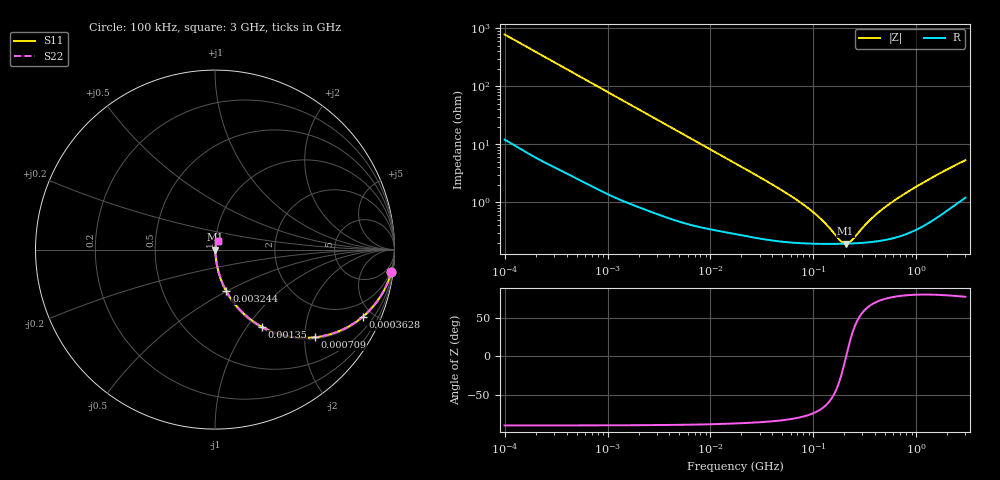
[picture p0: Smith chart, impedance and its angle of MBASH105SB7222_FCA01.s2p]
! MBASH105SB7222_FCA01  S-PARAMETER MODEL  ( Standard Model )
! Model Generated by TAIYO YUDEN Corporation (http://www.ty-top.com)
! Version 1.0
! TAIYO YUDEN Control No. 220601
! Copyright(c) 2019 TAIYO YUDEN CO.,LTD. All Rights Reserved.
! Product Description (link to TY-COMPAS)
! https://ds.yuden.co.jp/TYCOMPAS/or/detail?pn=MBASH105SB7222KFCA01&u=M
! Products Name : Multilayer Ceramic Capacitors
! Characteristics :
!  Capacitance : 2200 [pF] , Rated Voltage : 100 [V] , TCC : X7R
!  Case Size : 1.0 x 0.5 / 0.039 x 0.02 [mm/inch] , Thickness : 0.5 / 0.02 [mm/inch]
!  (Conditions: Temperature = 25 [degC] , DC Bias Voltage = 0 [V])
! External Node Assignments :
!  1  o---| |---o  2
! GND o---------o GND
! Frequency Range : 100kHz  -  3GHz  [ 401 STEP ]
# MHZ S RI R 50
! Freq[MHz].  S11 Real  S11 Imag  S21 Real  S21 Imag  S12 Real  S12 Imag  S22 Real  S22 Imag
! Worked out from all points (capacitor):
!   401 points, 100 kHz to 3 GHz, reference 50 ohm
!   read as one part in series: C = 2.03 nF near 105.3 kHz
!   lowest |Z| = 194 mohm at 205.6 MHz (marker M1)
!   series resonance near 208 MHz, so ESL is about 290 pH
!   S11 on the Smith chart (normalised r, x): 100 kHz: 1, -16; 362.8 kHz: 1.07, -4.36; 709 kHz: 1.04, -2.24; 1.35 MHz: 1.02, -1.18; 3.244 MHz: 1.01, -0.50; 3 GHz: 1.02, +0.10
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0.1  0.982 -0.1255  0.018 0.1255  0.018 0.1255  0.982 -0.1255
0.21115  0.9295 -0.2486  0.0705 0.2486  0.0705 0.2486  0.9295 -0.2486
0.362777  0.822 -0.3747  0.178 0.3747  0.178 0.3747  0.822 -0.3747
0.562235  0.6632 -0.4645  0.3368 0.4645  0.3368 0.4645  0.6632 -0.4645
0.709011  0.5562 -0.4885  0.4438 0.4885  0.4438 0.4885  0.5562 -0.4885
0.965977  0.4069 -0.4827  0.5931 0.4827  0.5931 0.4827  0.4069 -0.4827
1.350433  0.2635 -0.4314  0.7365 0.4314  0.7365 0.4314  0.2635 -0.4314
2.039661  0.1393 -0.336  0.8607 0.336  0.8607 0.336  0.1393 -0.336
3.161081  0.0661 -0.2368  0.9339 0.2368  0.9339 0.2368  0.0661 -0.2368
3.243608  0.0632 -0.2316  0.9368 0.2316  0.9368 0.2316  0.0632 -0.2316
7.027689  0.0169 -0.1132  0.9831 0.1132  0.9831 0.1132  0.0169 -0.1132
17.7727  0.0049 -0.0457  0.9951 0.0457  0.9951 0.0457  0.0049 -0.0457
52.46276  0.00229 -0.0149  0.9977 0.0149  0.9977 0.0149  0.00229 -0.0149
97.38194  0.00198 -0.00671  0.998 0.00671  0.998 0.00671  0.00198 -0.00671
129.3002  0.00193 -0.00397  0.9981 0.00397  0.9981 0.00397  0.00193 -0.00397
180.7614  0.00192 -0.00113  0.9981 0.00113  0.9981 0.00113  0.00192 -0.00113
205.6221  0.00193 -9.07e-05  0.9981 9.07e-05  0.9981 9.07e-05  0.00193 -9.07e-05
233.9019  0.00195 0.000949  0.9981 -0.000949  0.9981 -0.000949  0.00195 0.000949
362.5028  0.00208 0.0047  0.9979 -0.0047  0.9979 -0.0047  0.00208 0.0047
547.5153  0.0024 0.00903  0.9976 -0.00903  0.9976 -0.00903  0.0024 0.00903
1249.01  0.00466 0.0228  0.9953 -0.0228  0.9953 -0.0228  0.00466 0.0228
3000  0.0144 0.0504  0.9856 -0.0504  0.9856 -0.0504  0.0144 0.0504
